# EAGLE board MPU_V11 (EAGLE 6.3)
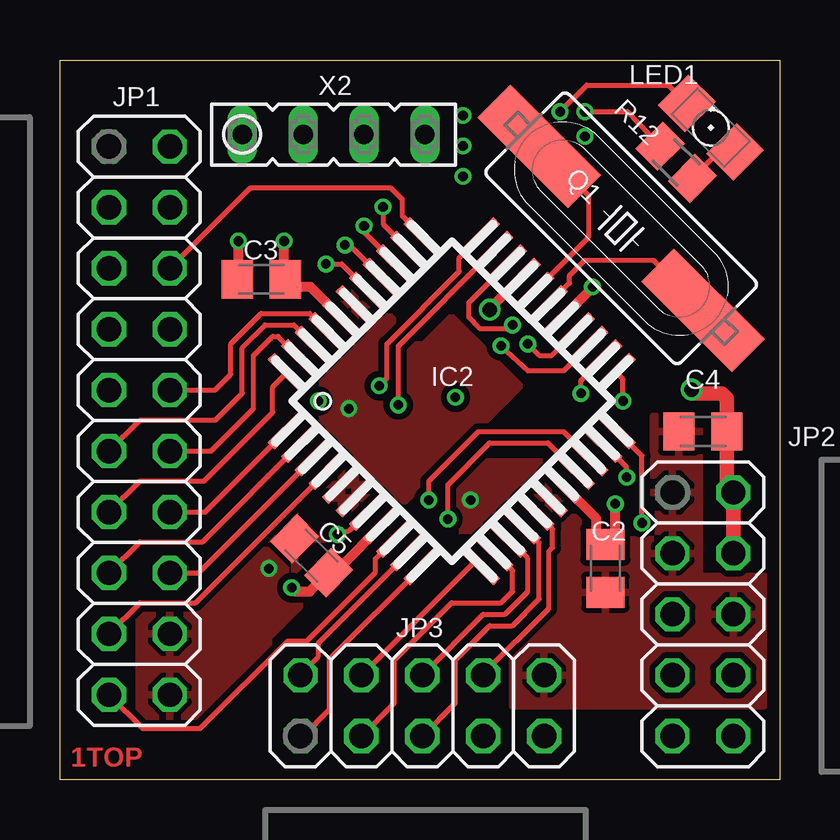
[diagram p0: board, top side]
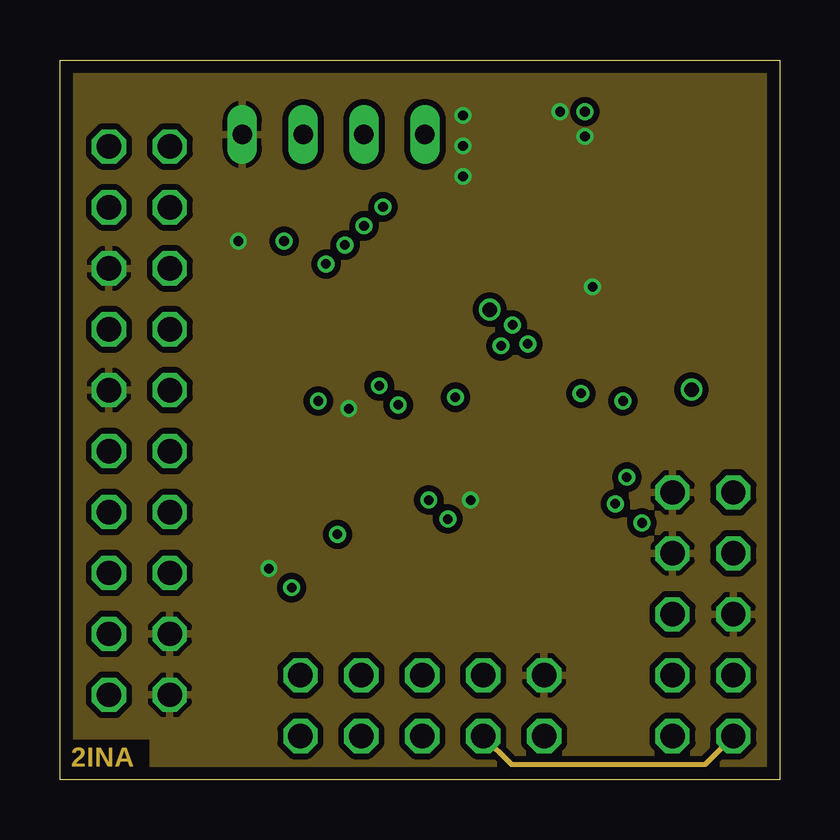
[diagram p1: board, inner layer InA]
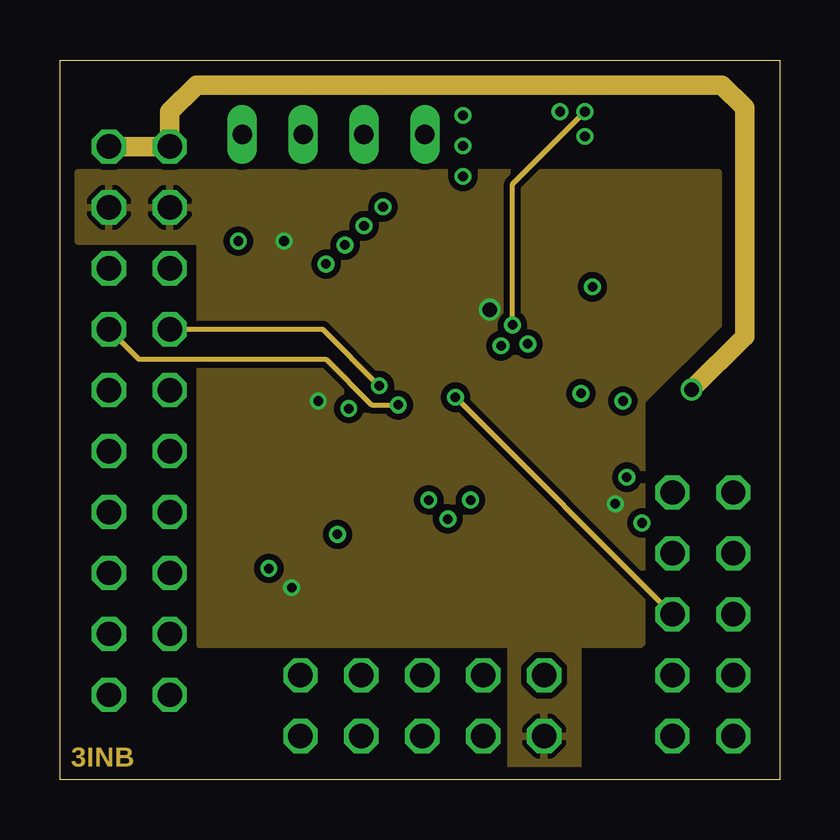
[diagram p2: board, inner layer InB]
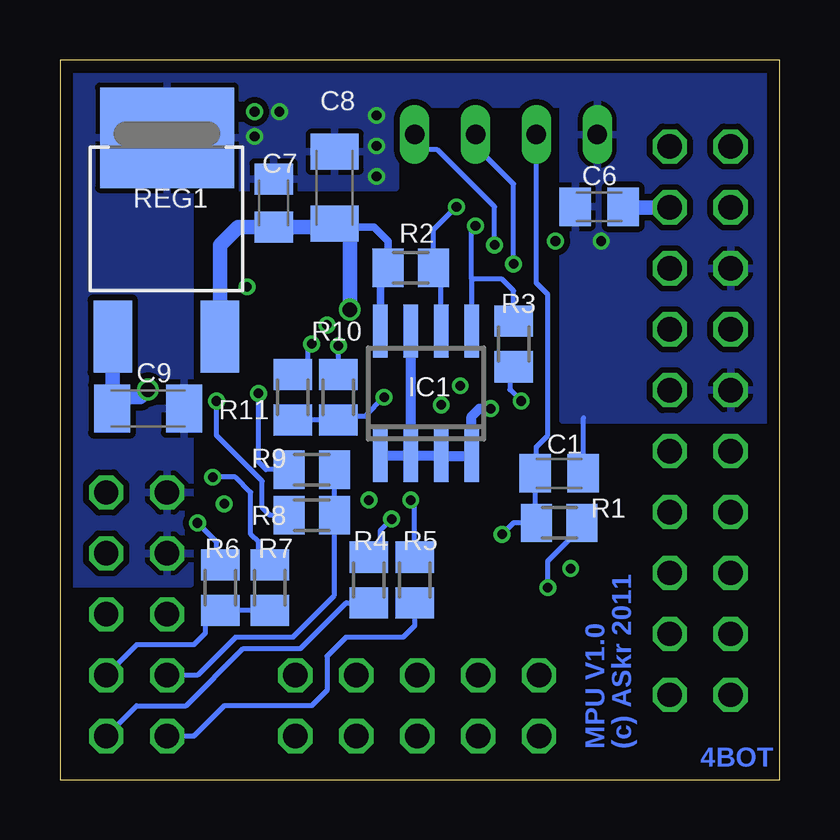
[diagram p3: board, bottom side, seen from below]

Size 30 x 30 mm. Coordinates in mm from the lower left corner, seen from the top.
Outline: 0,0 0,30 30,30 30,0 0,0
Copper layers (1*2+3*16): Top 0.035mm / dielectric 0.487mm / InA 0.035mm / dielectric 0.487mm / InB 0.035mm / dielectric 0.487mm / Bottom 0.035mm
Design rules "pcb-pool-2009 *": minimum track width 6mil, minimum drill 12mil, track to track 6mil, track to pad 6mil, pad to pad 6mil, via to via 6mil, smd to smd 6mil, copper to edge 20mil, drill to drill 8mil, minimum pad ring 8mil, minimum via ring 6mil, stop-mask expansion 3mil, vias tented up to drill 0mil, thermal gap 8mil

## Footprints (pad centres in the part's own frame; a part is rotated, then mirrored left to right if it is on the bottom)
C0805K = smd 1.3 x 1.6: 1 -1,0; 2 1,0
C1206K = smd 1.5 x 2: 1 -1.5,0; 2 1.5,0
AKKI_SOIC8 = smd 0.6 x 2.2: 1 -1.905,-2.6; 2 -0.635,-2.6; 3 0.635,-2.6; 4 1.905,-2.6; 5 1.905,2.6; 6 0.635,2.6; 7 -0.635,2.6; 8 -1.905,2.6
AKKI_P8X32A-Q44 = smd 1.9 x 0.4: 1 -5.713,4.013; 2 -5.713,3.212; 3 -5.713,2.413; 4 -5.713,1.613; 5 -5.713,0.812; 6 -5.713,0.013; 7 -5.713,-0.787; 8 -5.713,-1.587; 9 -5.713,-2.388; 10 -5.713,-3.188; 11 -5.713,-3.987; 23 5.688,-3.987; 24 5.688,-3.188; 25 5.688,-2.388; 26 5.688,-1.587; 27 5.688,-0.787; 28 5.688,0.013; 29 5.688,0.812; 30 5.688,1.613; 31 5.688,2.413; 32 5.688,3.212; 33 5.688,4.013 | smd 0.4 x 1.9: 12 -4.013,-5.688; 13 -3.212,-5.688; 14 -2.413,-5.688; 15 -1.613,-5.688; 16 -0.812,-5.688; 17 -0.013,-5.688; 18 0.787,-5.688; 19 1.587,-5.688; 20 2.388,-5.688; 21 3.188,-5.688; 22 3.987,-5.688; 34 3.987,5.713; 35 3.188,5.713; 36 2.388,5.713; 37 1.587,5.713; 38 0.787,5.713; 39 -0.013,5.713; 40 -0.812,5.713; 41 -1.613,5.713; 42 -2.413,5.713; 43 -3.212,5.713; 44 -4.013,5.713
2X10 = drill 1.016 octagon: 1 -11.43,-1.27; 2 -11.43,1.27; 3 -8.89,-1.27; 4 -8.89,1.27; 5 -6.35,-1.27; 6 -6.35,1.27; 7 -3.81,-1.27; 8 -3.81,1.27; 9 -1.27,-1.27; 10 -1.27,1.27; 11 1.27,-1.27; 12 1.27,1.27; 13 3.81,-1.27; 14 3.81,1.27; 15 6.35,-1.27; 16 6.35,1.27; 17 8.89,-1.27; 18 8.89,1.27; 19 11.43,-1.27; 20 11.43,1.27
2X05 = drill 1.016 octagon: 1 -5.08,-1.27; 2 -5.08,1.27; 3 -2.54,-1.27; 4 -2.54,1.27; 5 0,-1.27; 6 0,1.27; 7 2.54,-1.27; 8 2.54,1.27; 9 5.08,-1.27; 10 5.08,1.27
1206 = smd 1.6 x 1.803: A -1.422,0; C 1.422,0
AKKI_HC49UP = smd 5.334 x 1.93: 1 -4.826,0; 2 4.826,0
M0805 = smd 1.3 x 1.6: 1 -0.95,0; 2 0.95,0
AKKI_DPAK = smd 1.6 x 2.997: 1 -2.261,-4.928; 3 2.21,-4.928 | smd 5.588 x 4.191: 4 0,3.353
AKKI_FE04-1 = drill 0.813 long: 1 -5.08,0; 2 -2.54,0; 3 0,0; 4 2.54,0

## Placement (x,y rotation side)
C1  1n  [C0805K]  9.18,12.76 180 bottom
C2  100n  [C0805K]  22.74,8.81 90 top
C3  100n  [C0805K]  8.4,20.86 180 top
C4  100n  [C0805K]  26.8,14.51 180 top
C5  100n  [C0805K]  10.49,9.33 315 top
C6  100n  [C0805K]  7.52,23.88 180 bottom
C7  100n  [C0805K]  21.09,24.04 90 bottom
C8  22u;6V3  [C1206K]  18.55,24.67 90 bottom
C9  22u;6V3  [C1206K]  26.33,15.46 0 bottom
IC1  24LC256  [AKKI_SOIC8]  14.74,16.1 0 bottom
IC2  P8X32A-Q44  [AKKI_P8X32A-Q44]  16.35,15.78 45 top
JP1  [2X10]  3.31,14.96 270 top
JP2  [2X05]  26.8,6.89 270 top
JP3  [2X05]  15.11,3.08 0 top
LED1  green  [1206]  27.14,27.18 135 top
Q1  5.0-6.4MHz  [AKKI_HC49UP]  23.39,22.98 315 top
R1  470k  [M0805]  9.18,10.7 0 bottom
R2  18k  [M0805]  15.38,21.34 180 bottom
R3  18k  [M0805]  11.09,18.16 270 bottom
R4  240E  [M0805]  17.12,8.32 90 bottom
R5  240E  [M0805]  15.22,8.32 90 bottom
R6  240E  [M0805]  23.31,8 90 bottom
R7  470E  [M0805]  21.25,8 90 bottom
R8  470E  [M0805]  19.5,11.02 180 bottom
R9  240E  [M0805]  19.5,12.92 180 bottom
R10  470E  [M0805]  18.39,15.94 90 bottom
R11  240E  [M0805]  20.3,15.94 90 bottom
R12  470E  [M0805]  25.69,25.73 315 top
REG1  LF33  [AKKI_DPAK]  25.54,23.4 0 bottom
X2  [AKKI_FE04-1]  12.68,26.89 0 top

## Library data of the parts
C1-C7 = rcl
C8 C9 = rcl; SIZE: 1206
IC1 IC2 Q1 R1-R12 REG1 X2 = Akki
JP1-JP3 = pinhead
LED1 = led; SIZE: 1206

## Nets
!RES: C1.2 IC2.7 R1.1 X2.2
+3V3: C2.2 C3.1 C5.2 C6.1 C7.1 C8.1 IC1.8 IC2.8 IC2.18 IC2.30 IC2.40 JP1.3 JP1.4 JP3.9 R1.2 R2.2 R3.2 REG1.3
+UB: C4.1 C9.1 JP1.1 JP1.2 JP2.2 JP2.4 REG1.1
B: JP2.8 R6.1 R7.1
G: JP2.7 R8.1 R9.1
GND: C1.1 C2.1 C3.2 C4.2 C5.1 C6.2 C7.2 C8.2 C9.2 IC1.1 IC1.2 IC1.3 IC1.4 IC1.7 IC2.5 IC2.6 IC2.17 IC2.27 IC2.39 JP1.5 JP1.9 JP1.18 JP1.20 JP2.1 JP2.3 JP2.6 JP3.10 LED1.C REG1.4 X2.1
H: JP2.9 R5.1
N$1: IC2.28 Q1.2
N$2: IC2.29 Q1.1
N$3: IC2.38 X2.3
N$4: IC2.37 X2.4
N$5: IC2.19 R4.2
N$6: IC1.6 IC2.35 R2.1
N$7: IC1.5 IC2.36 R3.1
N$8: IC2.20 R5.2
N$9: IC2.22 R6.2
N$10: IC2.21 R7.2
N$11: IC2.23 R8.2
N$12: IC2.24 R9.2
N$13: IC2.26 R11.2
N$14: IC2.25 R10.2
N$15: LED1.A R12.2
P0: IC2.41 JP1.10
P1: IC2.42 JP1.11
P2: IC2.43 JP1.12
P3: IC2.44 JP1.13
P4: IC2.1 JP1.14
P5: IC2.2 JP1.15
P6: IC2.3 JP1.16
P7: IC2.4 JP1.17
P8: IC2.9 JP1.19
P9: IC2.10 JP3.2
P10: IC2.11 JP3.1
P11: IC2.12 JP3.4
P12: IC2.13 JP3.3
P13: IC2.14 JP3.6
P14: IC2.15 JP3.5
P15: IC2.16 JP3.8
P24: IC2.31 R12.1
P25: IC2.32 JP1.7
P26: IC2.33 JP1.8
P27: IC2.34 JP1.6
R: JP2.5 R10.1 R11.1
V: JP2.10 JP3.7 R4.1

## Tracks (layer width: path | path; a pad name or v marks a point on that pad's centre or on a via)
!RES  (via drill 0.4)
  Top 0.203: IC2.7 12.07,10.38 v11.56,10.22
  Bottom 0.203: v11.56,10.22 11.09,10.7 R1.1 10.18,10.75 C1.2 10.14,12.81 10.14,13.88 9.66,14.35 9.66,20.23 10.14,20.7 X2.2
+3V3  (via drill 0.4, 0.6)
  Top 0.406: IC2.8 11.67,8.85 C5.2 10.41,7.84 9.82,7.84 v9.66,8 | IC2.30 17.91,19.62 v17.91,19.59 | IC2.18 22.36,10.88 22.36,9.91 22.46,9.81 C2.2 22.9,9.81 23.15,10.06 v23.15,11.49 | v23.15,11.49 | IC2.40 10.43,20.54 9.98,20.54 9.66,20.86 C3.1 9.34,20.91 v9.34,22.45
  Bottom 0.203: 8.18,10.75 R1.2 8.23,10.54 9.66,9.11 v9.66,8 | R3.2 11.25,17.05 11.25,16.26 v10.77,15.78
  Bottom 0.305: IC1.8 16.64,21.02 R2.2 16.33,22.45 16.91,23.04 18.68,23.04
  Bottom 0.61: REG1.3 23.32,22.28 22.57,23.04 C7.1 18.68,23.04 C8.1 17.91,22.54 v17.91,19.59 | JP1.4 6.49,23.85 C6.1
  pour InB (isolate 0.254): 0.77,25.3 27.44,25.3 27.44,18.95 24.27,15.78 24.27,5.7 24.2,5.64 21.59,5.64 21.59,0.48 18.8,0.48 18.81,5.64 5.85,5.62 5.85,22.45 0.77,22.45
+UB  (via drill 0.6)
  Top 0.61: JP2.4 JP2.2 27.8,12.24 C4.1 27.8,15.89 27.6,16.1 26.49,16.1 v26.33,16.26
  InB 0.813: v26.33,16.26 28.55,18.48 28.55,28 27.6,28.96 5.69,28.96 4.58,27.84 JP1.2 JP1.1
  Bottom 0.61: v26.33,16.26 26.65,15.94 27.44,15.94 27.83,15.55 C9.1 27.8,15.5 REG1.1
B
  Bottom 0.203: JP2.8 26.8,5.62 24.42,5.62 23.95,6.1 23.95,6.73 23.79,6.89 23.47,6.89 R6.1 | R7.1 R6.1 | R6.1
G
  Bottom 0.203: R8.1 R9.1 | R8.1 | JP2.7 24.27,4.35 22.68,5.94 20.3,5.94 18.55,7.68 R8.1
GND  (via drill 0.4)
  Top 0.203: LED1.C 25.36,28.96 21.96,28.96 v20.85,27.84 | v20.85,27.84
  Top 0.406: IC2.27 22.2,20.51 v22.2,20.54 | C3.2 7.44,20.9 v7.44,22.45
  Bottom 0.203: C1.1 8.18,12.77 8.18,15.08
  Bottom 0.406: IC1.2 IC1.7 | IC1.2 IC1.1 | IC1.2 IC1.3 IC1.4 12.84,15.14 12.52,15.46 v12.04,15.46
  other vias: 8.71,8.79 17.12,11.65 16.8,25.15 16.8,26.42 16.8,27.69 21.88,26.81
  pour InA (isolate 0.254): 0.45,29.43 29.34,29.43 29.34,0.54 3.89,0.56 3.88,1.83 0.45,1.81
  pour Top (isolate 0.254): 16.33,13.24 24.74,13.24 24.74,15.14 26.65,15.14 26.65,8.48 29.34,8.48 29.34,3.08 18.87,3.08 18.87,10.38 16.33,10.38
  pour Top (isolate 0.254): 3.31,7.53 3.31,2.13 8.71,2.13 8.71,5.94 19.18,16.41 16.33,19.27 15.06,18 11.88,21.18 9.98,19.27 9.98,15.78 12.2,13.56 6.17,7.53
  pour Bottom (isolate 0.254): 24.58,8.16 29.66,8.16 29.66,29.75 0.45,29.75 0.45,14.99 9.03,14.99 9.03,28.16 16.01,28.16 16.01,24.67 24.58,24.67
H
  Bottom 0.203: R5.1 15.22,6.41 15.69,5.94 18.07,5.94 18.87,5.14 18.87,3.71 19.5,3.08 23.15,3.08 24.42,1.81 JP2.9
N$1
  Top 0.203: Q1.2 26.81,19.59 24.74,21.65 21.88,21.65 21.25,21.02 21.25,20.69 IC2.28
N$2
  Top 0.203: IC2.29 22.04,22.62 22.04,24.35 20,26.39 Q1.1
N$3  (via drill 0.4)
  Top 0.203: IC2.38 11.74,21.5 v11.09,21.5 | v11.09,21.5
  Bottom 0.203: X2.3 12.36,26.57 12.36,26.1 11.09,24.83 v11.09,21.5
N$4  (via drill 0.4)
  Top 0.203: IC2.37 12.08,22.29 v11.88,22.29
  Bottom 0.203: 14.9,26.42 14.9,26.57 X2.4 | 14.9,26.42 14.9,26.1 | v11.88,22.29 11.88,23.88 14.26,26.26 14.74,26.26 14.9,26.42
N$5  (via drill 0.4)
  Top 0.203: IC2.19 20.34,14.03 17.91,14.03 16.17,12.29 v16.17,10.86
  Bottom 0.203: R4.2 16.64,9.74 16.64,10.38 v16.17,10.86
N$6  (via drill 0.4)
  Top 0.203: IC2.35 13.47,23.16 v13.47,23.88
  Bottom 0.203: IC1.6 14.11,21.02 R2.1 14.43,22.92 v13.47,23.88
N$7  (via drill 0.4)
  Top 0.203: IC2.36 12.68,22.82 v12.68,23.08
  Bottom 0.203: 12.84,20.86 IC1.5 | 12.84,20.86 12.84,22.92 v12.68,23.08 | R3.1 11.09,20.38 11.56,20.86 12.84,20.86
N$8  (via drill 0.4)
  Top 0.203: IC2.20 20.99,14.51 17.44,14.51 15.38,12.45 v15.38,11.65
  Bottom 0.203: v15.38,11.65 15.22,11.49 R5.2
N$9  (via drill 0.4)
  Top 0.203: IC2.22 24.27,13.5 v24.27,10.7
  Bottom 0.203: R6.2 23.47,8.95 23.47,9.9 v24.27,10.7
N$10  (via drill 0.4)
  Top 0.203: v23.63,12.61 23.63,13 IC2.21
  Bottom 0.203: R7.2 21.73,9.43 21.73,9.91 22.04,10.22 22.04,11.97 22.68,12.61 v23.63,12.61
N$11  (via drill 0.4)
  Top 0.203: IC2.23 23.47,16.7 v23.47,15.78
  Bottom 0.203: v23.47,15.78 23.47,14.35 21.57,12.45 21.57,11.34 21.25,11.02 R8.2 | R8.2
N$12  (via drill 0.4)
  Top 0.203: IC2.24 21.73,16.64 v21.73,16.1
  Bottom 0.203: v21.73,16.1 21.73,13.24 21.41,12.92 R9.2
N$13  (via drill 0.4)
  Top 0.203: IC2.26 20.5,17.68 19.98,17.68 v19.5,18.16
  Bottom 0.203: v19.5,18.16 19.66,18 19.66,17.29 19.74,17.21 20.3,17.21 R11.2
N$14  (via drill 0.4)
  Top 0.203: IC2.25 21,17.05 19.5,17.05 | 19.5,17.05 | v18.39,18.08 19.5,17.05
  Bottom 0.203: R10.2 18.39,18.16 v18.39,18.08
N$15
  Top 0.203: R12.2 27.47,26.17 LED1.A
P0
  Top 0.203: JP1.10 6.46,16.23 7.12,16.89 7.12,18.16 8.39,19.43 10.41,19.43 IC2.41
P1
  Top 0.203: JP1.11 3.33,14.99 6.49,14.99 7.6,16.1 7.6,18 8.55,18.95 9.76,18.95 IC2.42
P2
  Top 0.203: JP1.12 6.3,13.69 8.07,15.46 8.07,17.68 8.87,18.48 9.1,18.48 IC2.43
P3
  Top 0.203: JP1.13 3.33,12.45 6.01,12.45 8.87,15.3 8.87,16.37 IC2.44
P4
  Top 0.203: JP1.14 6.05,11.15 IC2.1
P5
  Top 0.203: JP1.15 3.33,9.91 5.94,9.91 IC2.2
P6
  Top 0.203: JP1.16 5.78,8.61 IC2.3
P7
  Top 0.203: JP1.17 3.33,7.37 5.66,7.37 IC2.4
P8
  Top 0.203: IC2.9 13.15,9.2 13.15,8.64 10.29,5.78 9.5,5.78 5.85,2.13 3.44,2.13 JP1.19
P9
  Top 0.203: IC2.10 10.77,5.69 10.77,5.14 10.03,4.4 JP3.2
P10
  Top 0.203: IC2.11 11.25,5.03 11.25,2.92 10.14,1.81 JP3.1
P11
  Top 0.203: JP3.4 17.28,9.06 17.28,9.11 17.48,8.92 IC2.12
P12
  Top 0.203: JP3.3 13.95,3.19 13.95,4.99 16.33,7.37 18.39,7.37 18.87,7.84 18.87,8.71 IC2.13
P13
  Top 0.203: IC2.14 19.5,9.21 19.5,7.84 18.55,6.89 17.64,6.89 JP3.6
P14
  Top 0.203: JP3.5 16.49,3.19 16.49,4.99 17.91,6.41 18.87,6.41 19.98,7.53 19.98,9.87 IC2.15
P15
  Top 0.203: IC2.16 20.53,10.44 20.53,9.67 20.38,9.51 20.38,7.13 17.64,4.4 JP3.8
P24  (via drill 0.4)
  Top 0.203: IC2.31 17.04,19.88 17.04,19.27 17.52,18.8 18.55,18.8 v18.87,18.95 | v21.88,27.84 23.66,27.84 R12.1
  InB 0.203: v18.87,18.95 18.87,24.83 v21.88,27.84
P25  (via drill 0.4)
  Top 0.203: IC2.32 14.11,18.07 v14.11,15.62
  InB 0.203: v14.11,15.62 12.99,15.62 11.09,17.53 3.29,17.53 JP1.7
P26  (via drill 0.4)
  Top 0.203: IC2.33 16.64,21.75 16.64,21.18 13.63,18.16 13.63,16.73 v13.31,16.41
  InB 0.203: v13.31,16.41 10.95,18.77 JP1.8
P27
  Top 0.203: IC2.34 14.26,23.5 14.26,24.19 13.79,24.67 7.94,24.67 JP1.6
R  (via drill 0.4)
  InB 0.203: v16.49,15.94 JP2.5 | v16.49,15.94
  Bottom 0.203: R11.1 R10.1 18.23,15.14 17.28,15.14 v16.49,15.94 | v16.49,15.94
V
  InA 0.203: JP2.10 26.9,0.64 18.82,0.64 JP3.7
  Bottom 0.203: R4.1 18.07,7.37 19.98,5.46 22.36,5.46 24.74,3.08 26.8,3.08 JP2.10

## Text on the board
Top: 1TOP
InA: 2INA
InB: 3INB
Bottom: 4BOT | (c) ASkr 2011 | MPU V1.0
tDocu: GND | !RST | RX | TX | +UB | +UB | +3V3 | +3V3 | GND | P27 | P25 | P26 | GND | P0 | P1 | P2 | GND | +UB | P3 | P4 | GND | +UB | P5 | P6 | R | GND | P7 | GND | G | B | P8 | GND | H | V | P9 | P11 | P13 | P15 | GND | P10 | P12 | P14 | P16i | +3V3 | MicroPropUnit V1.1
bDocu: MicroPropUnit V1.1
